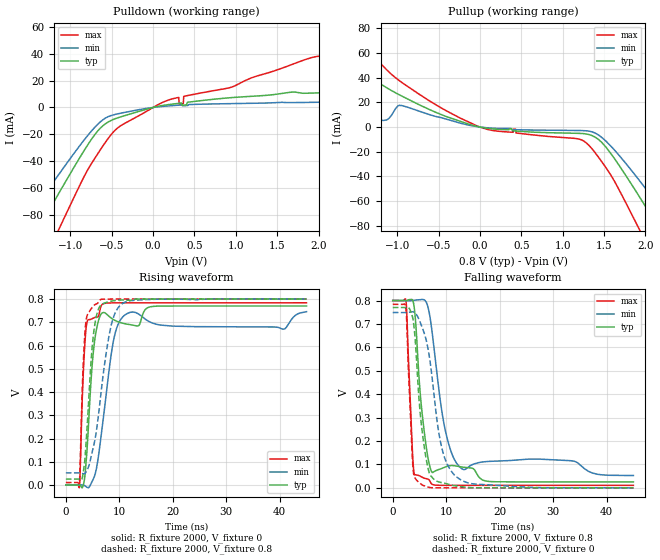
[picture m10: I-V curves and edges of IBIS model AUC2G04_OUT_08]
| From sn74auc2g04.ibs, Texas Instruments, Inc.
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[Model]   AUC2G04_OUT_08
Model_type  Output
Vref =   0
Rref =   2000
Cref =   15p
Vmeas =   0.4
| variable   typ   min   max
C_comp   5.67pF   2.72pF   7.64pF
| C_pullup   5.14pF   2.72pF   7.64pF
| C_pulldown   6.21pF   5.44pF   6.83pF
[Temperature Range]   40   100   -40
| Ambient temperature   25   85   -40
[Voltage range]   0.8   0.8   0.8
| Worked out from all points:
|   slope of the pulldown table from 0 to 0.12 V, typ, clamps not added: 77.1 ohm
|   slope of the pullup table from 0 to 0.12 V, typ, clamps not added: 92.7 ohm
|   rising waveform, R_fixture 2000, V_fixture 0: 20-80 % time 1.39ns typ, 2.47ns min, 816ps max; typ from 0 V to 0.77 V
|   falling waveform, R_fixture 2000, V_fixture 0.8: 20-80 % time 1.77ns typ, 2.85ns min, 868ps max; typ from 0.8 V to 0.026 V
|   rising waveform, R_fixture 2000, V_fixture 0.8: 20-80 % time 1.37ns typ, 2.65ns min, 763ps max; typ from 0.025 V to 0.8 V
|   falling waveform, R_fixture 2000, V_fixture 0: 20-80 % time 1.78ns typ, 2.86ns min, 866ps max; typ from 0.77 V to 0 V
[Pulldown]
| AUC2G04_OUT_08
|   Voltage   I(typ)   I(min)   I(max)
-3.6V     -332.2mA   -277.7mA   -406.7mA
-1.635V   -117.6mA   -94.23mA   -155.3mA
-1.375V   -89.31mA   -70.71mA   -121.6mA
-1.155V   -65.63mA   -51.24mA   -92.9mA
-630mV    -14.96mA   -10.34mA   -30.86mA
-430mV    -7.788mA   -4.786mA   -15.33mA
-90mV     -1.494mA   -794.3uA   -3.292mA
210mV     2.329mA    1.254mA    6.027mA
365mV     1.692mA    1.285mA    2.781mA
1.98V     10.83mA    3.867mA    38.03mA
2.365V    11.74mA    4.199mA    33.49mA
7.2V      23.85mA    8.894mA    59.33mA
[Pullup]
| AUC2G04_OUT_08
|   Voltage   I(typ)   I(min)   I(max)
-3.6V     79.22mA    9.067mA    184.4mA
-3.085V   77.82mA    9.388mA    162mA
-1.585V   27.55mA    10.91mA    82.21mA
-1.305V   38.3mA     6.636mA    59.53mA
-1.13V    31.96mA    5.757mA    46.56mA
-975mV    26.16mA    17.62mA    37.64mA
-235mV    4.613mA    3.12mA     7.149mA
1.36V     -7.061mA   -3.967mA   -18.08mA
1.87V     -50.4mA    -38.36mA   -75.46mA
2.115V    -76.54mA   -59.59mA   -107.8mA
2.4V      -107.5mA   -85.11mA   -145.4mA
7.2V      -634.1mA   -537.5mA   -765.5mA
[Ramp]
| AUC2G04_OUT_08
| variable   typ   min   max
dV/dt_r   0.47/1.41E-09   0.45/2.51E-09   0.48/8.21E-10
dV/dt_f   0.47/1.77E-09   0.45/2.85E-09   0.48/8.72E-10
R_load = 2000
[Rising Waveform]
| AUC2G04_OUT_08
R_fixture =   2000
C_fixture =   0
L_fixture =   0
V_fixture =   0
V_fixture_min = 0
V_fixture_max = 0
|   Time   V(typ)   V(min)   V(max)
0s        8.052nV    45.46nV    527.4pV
2.535ns   679uV      700.9uV    -9.242mV
3.38ns    11.54mV    -1.081mV   537.7mV
3.94ns    146.4mV    -9.284mV   698.6mV
5.2ns     585.6mV    29.44mV    718.6mV
6.825ns   740.8mV    253.9mV    777.7mV
9.03ns    709.8mV    634.5mV    783.5mV
11.37ns   692.3mV    736.5mV    783.6mV
40.67ns   770mV      670.2mV    783.8mV
45ns      770mV      745.5mV    783.8mV
[Falling Waveform]
| AUC2G04_OUT_08
R_fixture =   2000
C_fixture =   0
L_fixture =   0
V_fixture =   0.8
V_fixture_min = 0.8
V_fixture_max = 0.8
|   Time   V(typ)   V(min)   V(max)
0s        800mV      800mV      800mV
2.49ns    798.8mV    799.7mV    796.1mV
3.675ns   803mV      799.8mV    159.9mV
4.095ns   755.1mV    801.4mV    55.24mV
5.51ns    315.3mV    804.3mV    45.31mV
7.365ns   65.82mV    664.7mV    15.23mV
9.86ns    89.39mV    242.3mV    10.72mV
12.92ns   89.16mV    81.7mV     10.65mV
27.33ns   25.56mV    122.8mV    10.61mV
45ns      25.5mV     52.51mV    10.6mV
[Rising Waveform]
| AUC2G04_OUT_08
R_fixture =   2000
C_fixture =   0
L_fixture =   0
V_fixture =   0.8
V_fixture_min = 0.8
V_fixture_max = 0.8
|   Time   V(typ)   V(min)   V(max)
0s        25.46mV    52.25mV    10.6mV
2.515ns   25.31mV    52.14mV    8.832mV
3.115ns   35.13mV    49.36mV    441.8mV
3.53ns    104.2mV    49.43mV    641.3mV
3.885ns   217mV      60.32mV    720.8mV
5.07ns    628.6mV    155.9mV    767.8mV
6.41ns    770mV      363mV      796.7mV
8.515ns   790.7mV    690.6mV    799.8mV
10.88ns   795.9mV    784.8mV    799.9mV
45ns      800mV      800mV      800mV
[Falling Waveform]
| AUC2G04_OUT_08
R_fixture =   2000
C_fixture =   0
L_fixture =   0
V_fixture =   0
V_fixture_min = 0
V_fixture_max = 0
|   Time   V(typ)   V(min)   V(max)
0s        770mV      748.6mV    783.8mV
2.415ns   769.7mV    748.5mV    775.6mV
2.59ns    770.2mV    748.6mV    722.9mV
3.005ns   769.1mV    749.5mV    466.4mV
3.815ns   716.1mV    751.6mV    79.9mV
5.23ns    297.4mV    701.2mV    17.16mV
6.97ns    55.88mV    541.4mV    1.236mV
9.125ns   22.46mV    175.4mV    97.74uV
12.04ns   7.32mV     44.69mV    49.73uV
45ns      27.3uV     2.571uV    8.329uV
